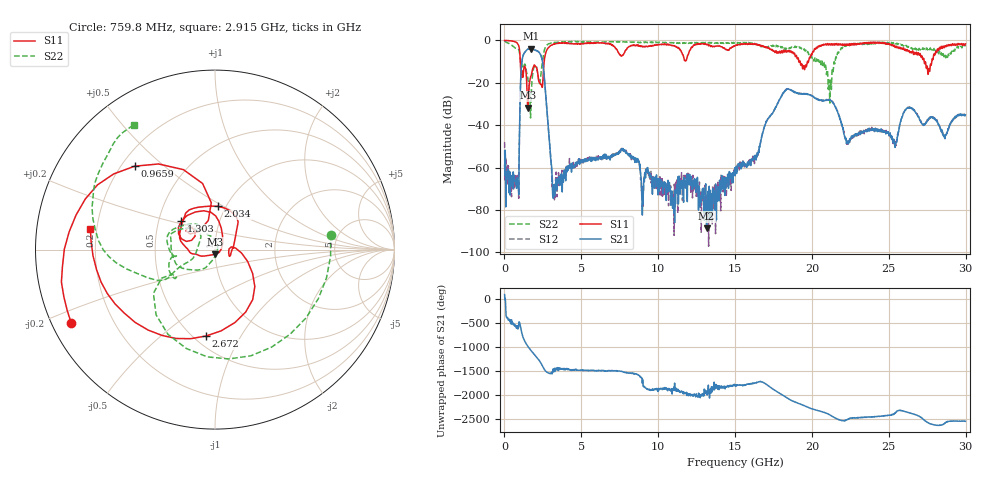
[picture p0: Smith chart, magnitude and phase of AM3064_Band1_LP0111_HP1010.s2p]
# Hz S DB R 50.0
!freq dBS11 angS11 dBS21 angS21 dBS12 angS12 dBS22 angS22
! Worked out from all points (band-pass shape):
!   1600 points, 10 MHz to 29.98 GHz, reference 50 ohm
!   highest |S21| = -3.99 dB at 1.716 GHz (marker M1); lowest = -88.7 dB at 13.15 GHz (marker M2)
!   |S21| within 3 dB of the highest: 1.223 GHz to 2.361 GHz (1.138 GHz wide, 63.5 % of centre)
!   lowest |S11| = -31.7 dB at 1.528 GHz (marker M3), VSWR 1.05, Z = 50.1 - j2.59 ohm
!   |S11| at or under -10 dB: 1.031 GHz to 2.584 GHz (1.553 GHz wide, 85.9 % of centre); 19.23 GHz to 19.7 GHz (472.4 MHz wide, 2.43 % of centre); 27.3 GHz to 27.79 GHz (491.6 MHz wide, 1.78 % of centre)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
!   |S22| runs from -36.6 to -0.3 dB; largest |S21 - S12| = 0.0084
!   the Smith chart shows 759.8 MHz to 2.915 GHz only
!   S11 on the Smith chart (normalised r, x): 759.8 MHz: 0.06, -0.24; 965.9 MHz: 0.25, +0.40; 1.303 GHz: 0.66, +0.22; 2.034 GHz: 0.92, +0.47; 2.672 GHz: 0.58, -0.72; 2.915 GHz: 0.17, +0.08
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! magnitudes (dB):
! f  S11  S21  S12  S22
! 10 MHz  0.0  -58.9  -48.1  -0.3
! 759.8 MHz  -0.9  -66.5  -64.1  -3.7
! 965.9 MHz  -3.8  -48.8  -48.8  -5.4
! 1.303 GHz  -12.2  -5.9  -5.8  -11.3
! 1.528 GHz  -31.7  -4.2  -4.1  -18.3
! 1.716 GHz  -16.9  -4.0  -4.0  -34.1
! 2.034 GHz  -12.3  -4.8  -4.7  -11.7
! 2.672 GHz  -6.3  -24.5  -24.4  -3.1
! 2.915 GHz  -3.0  -46.9  -46.5  -1.6
! 3.271 GHz  -1.7  -70.5  -69.1  -0.9
! 5.015 GHz  -1.5  -56.5  -55.8  -0.7
! 7.732 GHz  -6.7  -51.4  -51.4  -0.7
! 10 GHz  -2.1  -66.5  -68.6  -1.0
! 13.15 GHz  -2.1  -88.7  -76.1  -1.2
! 15 GHz  -2.6  -63.9  -60.4  -1.4
! 18.25 GHz  -5.0  -23.7  -23.7  -4.3
! 19.99 GHz  -6.8  -26.2  -26.1  -7.9
! 21.17 GHz  -2.0  -28.1  -28.0  -29.6
! 22.32 GHz  -2.0  -47.5  -48.1  -2.6
! 25 GHz  -1.5  -44.2  -43.9  -1.1
! 27.56 GHz  -16.0  -37.2  -36.8  -3.7
! 29.98 GHz  -1.7  -35.2  -35.4  -2.8
